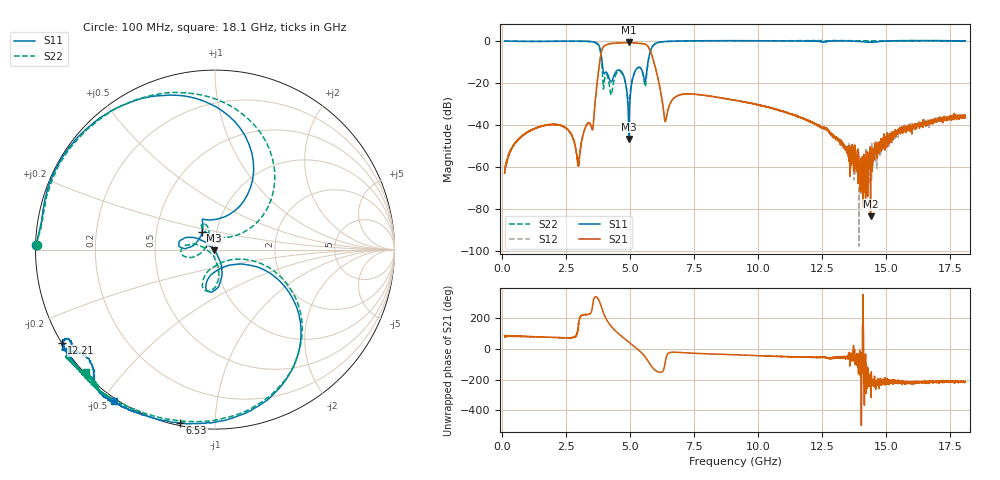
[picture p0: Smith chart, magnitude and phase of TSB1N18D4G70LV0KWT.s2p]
! TSB1N18D4G70LV0KWT  S-PARAMETER MODEL  ( General Type )
! Model Generated by TAIYO YUDEN Corporation (https://www.yuden.co.jp/en/)
! Version 1.0
! TAIYO YUDEN Control No. 20240527
! Copyright(c) 2024 TAIYO YUDEN CO.,LTD. All Rights Reserved.
! Products Name : Ceramic RF Devices
! Characteristics :
!  Passband freq : 4400-5000MHz ( At Passband , Insertion Loss : 1.6dB , VSWR 2.0 )
!  Attenuation : 35 dB min at 500to 3300MHz, 20 dB min at 6450to 7700MHz, Impedance : 50 Ohm
!  Case Size : 1.6 x 0.8 / 0.063 x 0.031 [mm/inch] , Thickness : 0.65/ 0.026 [mm/inch]
!  (Conditions: Temperature = 25 degC , DC Bias Current/Voltage = 0A / 0V)
! External Node Assignments :
!  1  o---|-------|---o  2
!  |  BPF  |
! GND o---|-------|---o GND
! Frequency Range : 100MHz  -  18.1GHz  [ 3601 STEP ]
# MHZ S RI R 50
! Freq[MHz].  S11 Real  S11 Imag  S21 Real  S21 Imag  S12 Real  S12 Imag  S22 Real  S22 Imag
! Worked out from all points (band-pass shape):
!   3601 points, 100 MHz to 18.1 GHz, reference 50 ohm
!   highest |S21| = -0.70 dB at 4.94 GHz (marker M1); lowest = -83.3 dB at 14.39 GHz (marker M2)
!   |S21| within 3 dB of the highest: 3.92 GHz to 5.756 GHz (1.837 GHz wide, 38 % of centre)
!   lowest |S11| = -46.6 dB at 4.95 GHz (marker M3), VSWR 1.01, Z = 49.6 - j0.18 ohm
!   |S11| at or under -10 dB: 3.909 GHz to 5.702 GHz (1.792 GHz wide, 37.3 % of centre)
!   |S22| runs from -30.3 to 0.3 dB; largest |S21 - S12| = 0.0046
!   S11 on the Smith chart (normalised r, x): 100 MHz: 0.00, +0.01; 4.2 GHz: 0.85, +0.17; 6.53 GHz: 0.01, -0.82; 12.21 GHz: 0.00, -0.28; 18.1 GHz: -0.01, -0.53
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100  -0.9949 0.0275  1.34e-05 0.000714  0.000128 0.000728  -0.9928 0.0279
1435  -0.9602 0.2005  0.00161 0.00878  0.00168 0.00898  -0.9546 0.2059
2965  -0.8735 0.475  -0.000874 0.000771  -0.00101 0.000717  -0.8454 0.5088
3100  -0.8427 0.5273  -0.00317 -0.00242  -0.00309 -0.00239  -0.8075 0.5657
3540  -0.5645 0.7798  0.00212 -0.00752  0.00218 -0.00756  -0.4627 0.8253
3940  0.0824 0.197  -0.3048 -0.6245  -0.304 -0.6245  0.0793 0.0694
4200  -0.0722 0.0979  -0.8175 0.2648  -0.8172 0.2644  -0.0324 0.077
4665  -0.1774 0.06  0.1001 0.9009  0.0988 0.8993  -0.1756 0.0142
4940  -0.0115 0.00456  0.6345 0.6693  0.6323 0.6689  -0.0255 -0.0182
4950  -0.00431 -0.00181  0.6497 0.6537  0.6471 0.6528  -0.0207 -0.0227
5225  0.0204 -0.2054  0.883 0.1302  0.8821 0.1311  0.00236 -0.2071
5640  0.1418 -0.0801  0.3739 -0.7198  0.3737 -0.7179  0.1312 -0.053
6100  0.1707 -0.9119  -0.1059 -0.0623  -0.105 -0.0622  0.1691 -0.9011
6355  -0.0841 -0.9701  -0.00351 -0.0129  -0.00352 -0.0128  -0.0966 -0.9598
6530  -0.1937 -0.9664  0.0259 -0.0118  0.0261 -0.0122  -0.2136 -0.9512
9100  -0.6215 -0.8075  0.0309 -0.0238  0.0304 -0.0238  -0.6536 -0.7756
12100  -0.8491 -0.5232  0.00694 -0.0095  0.00667 -0.00962  -0.8223 -0.6064
12210  -0.8542 -0.5192  0.0064 -0.00892  0.00658 -0.00892  -0.8242 -0.6
14040  -0.7819 -0.5665  -9.3e-05 -0.000262  0.00108 0.000355  -0.7808 -0.637
14395  -0.7047 -0.6072  -6.46e-05 -2.24e-05  -0.00259 -0.000432  -0.7678 -0.658
15100  -0.6688 -0.7471  -0.00499 0.00266  -0.00423 0.00343  -0.7202 -0.6954
18100  -0.5621 -0.8422  -0.0133 0.00796  -0.0142 0.00965  -0.7193 -0.6797
